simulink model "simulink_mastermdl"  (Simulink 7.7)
settings: Solver=ode45  StartTime=0.0  StopTime=86400  RelTol=1e-3
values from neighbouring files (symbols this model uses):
  To = 273+0    (= 273)    [model_master_simulink_floor.m]    (also in model_master_simulink_PI_tuning.m; model_master_simulink_storing_floorroom.m; sfunctionmodel.m = u(3); equations.m = d(1))

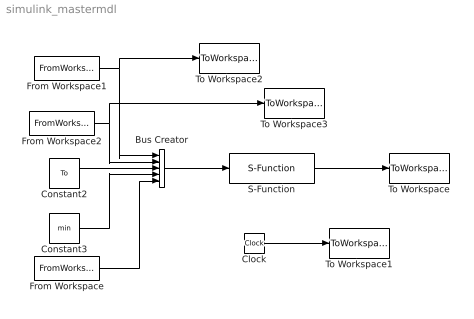
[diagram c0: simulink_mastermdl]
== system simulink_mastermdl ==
  Bus Creator : BusCreator  Inputs=5
  Clock : Clock
  Constant2 : Constant  Value=To
  Constant3 : Constant  Value=min
  From Workspace : FromWorkspace  VariableName=var  SampleTime=0
  From Workspace1 : FromWorkspace  VariableName=varqhf  SampleTime=0
  From Workspace2 : FromWorkspace  VariableName=varqhr  SampleTime=0
  S-Function : S-Function  FunctionName=sfunctionmodel  Parameters=init, par, var  EnableBusSupport=off
  To Workspace : ToWorkspace  VariableName=simout  SampleTime=-1  SaveFormat=Array
  To Workspace1 : ToWorkspace  VariableName=time  SampleTime=-1  SaveFormat=Array
  To Workspace2 : ToWorkspace  VariableName=qhf_out  SampleTime=-1  SaveFormat=Array
  To Workspace3 : ToWorkspace  VariableName=qhr_out  SampleTime=-1  SaveFormat=Array
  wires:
  Constant2/1 -> Bus Creator/3
  Constant3/1 -> Bus Creator/4
  Bus Creator/1 -> S-Function/1
  S-Function/1 -> To Workspace/1
  Clock/1 -> To Workspace1/1
  From Workspace1/1 -> Bus Creator/1, To Workspace2/1
  From Workspace2/1 -> Bus Creator/2, To Workspace3/1
  From Workspace/1 -> Bus Creator/5
